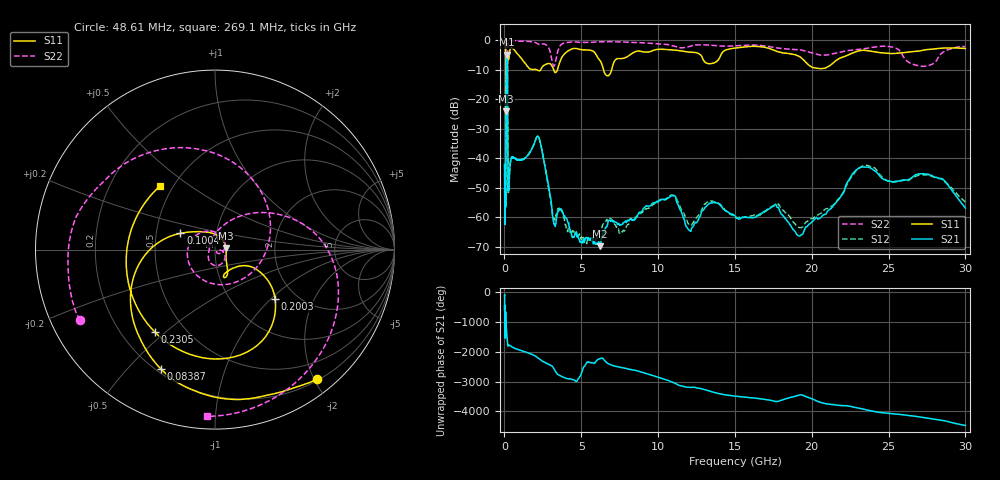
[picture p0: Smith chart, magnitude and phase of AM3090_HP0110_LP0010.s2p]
! Date/Time: Thu, Feb 28, 2019 1:59 PM
! Network Analyzer: Agilent Technologies E8364B Rev: A.07.50.67
! Sweep from 0.010 to 30.000 GHz, 1601 Points, Sweep Type: LOG
! Power Supply: 5.023 V, 0.002 A
# Hz S DB R 50
!freq MagS11 AngS11 MagS21 AngS21 MagS12 AngS12 MagS22 AngS22
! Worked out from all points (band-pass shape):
!   1601 points, 10 MHz to 30 GHz, reference 50 ohm
!   highest |S21| = -4.99 dB at 144.7 MHz (marker M1); lowest = -69.7 dB at 6.202 GHz (marker M2)
!   |S21| within 3 dB of the highest: 109.3 MHz to 185.1 MHz (75.78 MHz wide, 51.5 % of centre)
!   lowest |S11| = -24.2 dB at 107.7 MHz (marker M3), VSWR 1.13, Z = 56.5 + j0.981 ohm
!   |S11| at or under -10 dB: 2.064 GHz to 2.362 GHz (297.5 MHz wide, 13.4 % of centre); 3.198 GHz to 3.452 GHz (254.2 MHz wide, 7.65 % of centre); 6.447 GHz to 6.978 GHz (531.5 MHz wide, 7.92 % of centre)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
!   |S22| runs from -37.1 to -0.2 dB; largest |S21 - S12| = 0.012
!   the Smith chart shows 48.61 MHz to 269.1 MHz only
!   S11 on the Smith chart (normalised r, x): 48.61 MHz: 0.23, -2.05; 83.87 MHz: 0.22, -0.62; 100.4 MHz: 0.67, +0.13; 200.3 MHz: 1.57, -1.06; 230.5 MHz: 0.34, -0.46; 269.1 MHz: 0.43, +0.38
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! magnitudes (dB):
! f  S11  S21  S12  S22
! 10 MHz  -0.2  -42.0  -42.1  -0.5
! 38.04 MHz  -0.5  -59.3  -59.0  -1.3
! 48.61 MHz  -0.8  -48.2  -48.6  -1.5
! 75.5 MHz  -1.8  -56.6  -54.9  -3.7
! 83.87 MHz  -2.7  -48.1  -48.9  -5.8
! 100.4 MHz  -13.4  -15.3  -15.3  -15.1
! 107.7 MHz  -24.2  -8.7  -8.7  -17.9
! 134.2 MHz  -16.1  -5.1  -5.1  -36.9
! 144.7 MHz  -16.9  -5.0  -5.0  -26.8
! 178.6 MHz  -14.8  -6.7  -6.7  -29.5
! 200.3 MHz  -7.3  -18.8  -18.7  -9.3
! 230.5 MHz  -4.9  -50.7  -49.3  -1.5
! 269.1 MHz  -6.6  -50.8  -50.7  -0.6
! 550.5 MHz  -3.0  -39.7  -39.7  -0.2
! 2.084 GHz  -10.0  -33.0  -33.0  -1.0
! 3.236 GHz  -10.5  -62.3  -60.6  -8.8
! 6.202 GHz  -6.8  -69.7  -64.5  -0.6
! 7.926 GHz  -5.8  -61.7  -63.1  -0.7
! 10.76 GHz  -3.3  -53.1  -52.6  -1.7
! 19.31 GHz  -6.0  -65.9  -63.5  -3.4
! 23.48 GHz  -3.5  -43.0  -42.4  -2.9
! 30 GHz  -2.9  -56.9  -54.8  -2.2
